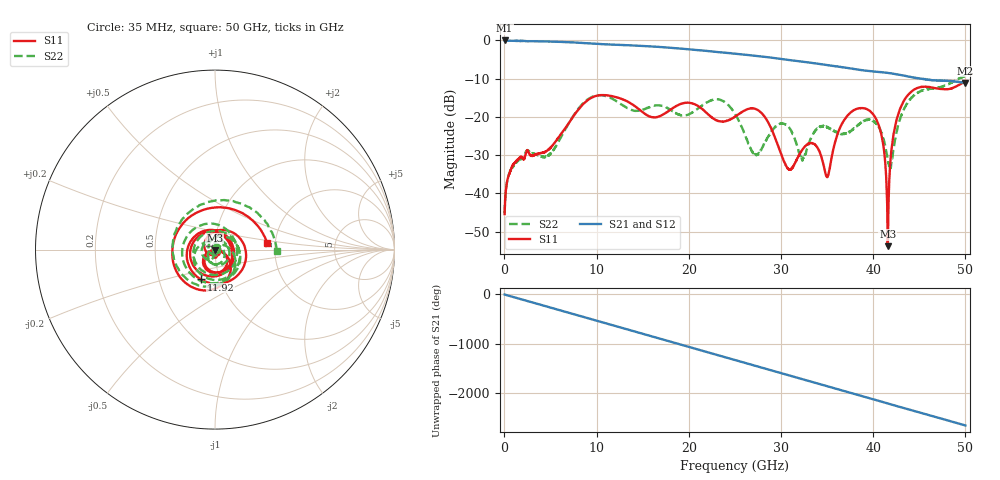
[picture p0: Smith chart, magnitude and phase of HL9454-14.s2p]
! 3/7/2022 11:44:47 AM
! H:\PRODUCTION_DATA\TEMP_S2P.S2P
! CHANNEL.1
! TR.MEASUREMENT
! CORRECTED.DATA
# GHZ S RI R 50.0
! FREQ.GHZ  S11RE  S11IM  S21RE  S21IM  S12RE  S12IM  S22RE  S22IM
!; PortSelection: Port_12
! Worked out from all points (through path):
!   3571 points, 35 MHz to 50 GHz, reference 50 ohm
!   highest |S21| = -0.03 dB at 35 MHz (marker M1); lowest = -11.1 dB at 49.99 GHz (marker M2)
!   group delay of S21, straight-line fit = 148 ps
!   lowest |S11| = -53.8 dB at 41.57 GHz (marker M3), VSWR 1.00, Z = 49.9 - j0.167 ohm
!   |S11| at or under -10 dB: start of sweep to end of sweep
!   |S22| runs from -45.3 to -9.2 dB; largest |S21 - S12| = 0.0095
!   S11 on the Smith chart (normalised r, x): 35 MHz: 1.01, +0.01; 11.92 GHz: 0.81, -0.28; 50 GHz: 1.81, +0.14
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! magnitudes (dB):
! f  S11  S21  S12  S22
! 35 MHz  -45.4  0.0  0.0  -45.3
! 1.113 GHz  -32.0  -0.1  -0.1  -32.3
! 4.906 GHz  -28.3  -0.3  -0.3  -29.9
! 8.376 GHz  -17.1  -0.7  -0.6  -16.9
! 11.92 GHz  -14.7  -1.1  -1.1  -15.5
! 16.7 GHz  -19.9  -1.7  -1.7  -17.0
! 19.88 GHz  -16.3  -2.3  -2.3  -19.5
! 25.03 GHz  -19.9  -3.5  -3.5  -19.2
! 27.21 GHz  -17.9  -4.0  -4.0  -29.7
! 30.83 GHz  -33.6  -5.1  -5.1  -22.6
! 32.31 GHz  -28.6  -5.6  -5.6  -31.4
! 33.36 GHz  -26.9  -5.9  -5.9  -25.0
! 35.02 GHz  -35.7  -6.5  -6.4  -22.8
! 36.86 GHz  -20.8  -7.1  -7.1  -24.5
! 39.55 GHz  -18.3  -8.0  -8.0  -20.7
! 40.87 GHz  -24.5  -8.3  -8.4  -24.1
! 41.57 GHz  -53.8  -8.5  -8.5  -31.2
! 41.69 GHz  -40.8  -8.5  -8.6  -32.1
! 42.29 GHz  -23.5  -8.8  -8.8  -27.3
! 43.53 GHz  -15.0  -9.3  -9.3  -17.1
! 49.99 GHz  -10.7  -11.1  -11.1  -9.3
! 50 GHz  -10.7  -11.1  -11.1  -9.2
